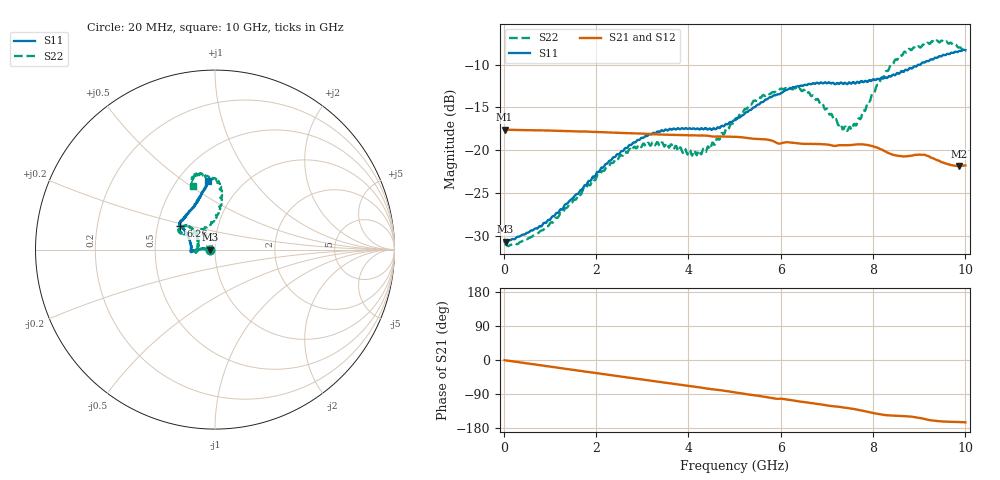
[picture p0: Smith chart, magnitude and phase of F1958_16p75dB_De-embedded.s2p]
! Integrated Device Technology
! Corporate Headquarters
! 6024 Silver Creek Valley Road
! San Jose, CA 95138  USA
! Phone:  1-408-284-8200
! Toll Free:  1-800-223-1366
! Webpage:  http://www.idt.com/
! Timing and RF Division
! 515 Groton Road, Suite 102
! Westford, MA 01886-6024
! Device:  F1958
! Description: 7-bit 0.25 dB Digital Step Attenuator
! Frequency:  0.001 -  6.000 GHz
! Package:  4x4 mm Thin QFN Plastic Package: 24 pin
! Ports:  2 RF, 12 DC
!  Pin  1  = D0
!  Pin  2  = VDD
!  Pin  3  = VMODE
!  Pin  4  = GND
!  Pin  5  = RF1  =  Port 1
!  Pin  6  = GND
!  Pin  7  = GND
!  Pin  8  = GND
!  Pin  9  = GND
!  Pin 10  = GND
!  Pin 11  = GND
!  Pin 12  = GND
!  Pin 13  = GND
!  Pin 14  = RF2  =  Port 2
!  Pin 15  = GND
!  Pin 16  = LE
!  Pin 17  = CLK
!  Pin 18  = DATA
!  Pin 19  = D6
!  Pin 20  = D5
!  Pin 21  = D4
!  Pin 22  = D3
!  Pin 23  = D2
!  Pin 24  = D1
! State:  67
! Atten State:  16.75 dB
! Voltage:  +3.30 Volts
! Current:  0.258 mA
! Data:  The device was measured on a F1958 evaluation board which has
!  individual transmission lines to the RF pins.  Data was collected
!  using a calibrated network analyzer.  The evaluation board was
!  de-embedded using Automatic Fixture Removal (AFR).
!  The reference plane is the edge of the package pin.
! Misc:
!  Action Tracker AT0419
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# GHz S dB R 50
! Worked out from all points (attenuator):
!   500 points, 20 MHz to 10 GHz, reference 50 ohm
!   highest |S21| = -17.58 dB at 20 MHz (marker M1); lowest = -21.8 dB at 9.86 GHz (marker M2)
!   lowest |S11| = -30.6 dB at 40 MHz (marker M3), VSWR 1.06, Z = 47.1 - j0.0698 ohm
!   |S11| at or under -10 dB: start of sweep to 9.027 GHz
!   |S22| runs from -31.1 to -7.2 dB; largest |S21 - S12| = 0.00044
!   S11 on the Smith chart (normalised r, x): 20 MHz: 0.94, -0.00; 6.26 GHz: 0.66, +0.18; 10 GHz: 0.69, +0.62
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0.02  -30.61 -178.5  -17.58 -0.5  -17.57 -0.4  -30.98 -178.7
0.04  -30.64 -178.6  -17.59 -0.8  -17.58 -0.8  -30.94 -178.2
0.32  -30.04 177.5  -17.62 -5.7  -17.62 -5.7  -30.84 177.1
0.84  -28.68 175.6  -17.67 -14.6  -17.67 -14.6  -29.30 176.6
1.7  -24.55 176.3  -17.80 -29.3  -17.79 -29.3  -24.78 175.4
2.62  -19.80 -179.8  -17.98 -44.9  -17.96 -45.0  -20.17 -178.4
2.92  -18.77 -177.1  -18.03 -50.0  -18.02 -50.1  -19.35 -175.8
3.36  -17.85 -174.7  -18.14 -57.6  -18.14 -57.7  -19.33 -171.4
4.24  -17.57 -179.9  -18.26 -72.3  -18.27 -72.3  -20.04 166.7
4.5  -17.61 174.2  -18.37 -77.0  -18.38 -77.1  -19.42 151.5
5.02  -16.47 159.9  -18.42 -85.7  -18.43 -85.7  -16.28 138.5
5.54  -14.62 149.8  -18.67 -94.9  -18.68 -94.9  -13.85 139.8
6.26  -12.65 145.8  -19.11 -106.9  -19.12 -106.9  -12.90 150.6
6.68  -12.22 143.7  -19.25 -113.7  -19.26 -113.6  -13.65 153.0
7.3  -12.09 137.2  -19.39 -124.2  -19.40 -124.0  -16.91 132.2
7.5  -12.13 134.3  -19.39 -127.7  -19.39 -127.6  -17.25 114.3
7.7  -12.16 130.2  -19.29 -132.0  -19.29 -132.0  -16.25 98.0
8.34  -11.36 115.3  -20.31 -146.2  -20.32 -146.3  -10.59 82.6
8.68  -10.74 108.6  -20.69 -148.2  -20.69 -148.1  -8.49 87.0
9.26  -9.37 100.8  -20.85 -159.2  -20.85 -159.2  -7.38 99.6
9.86  -8.44 96.2  -21.82 -163.6  -21.85 -163.6  -8.03 108.2
10  -8.33 96.1  -21.74 -164.6  -21.79 -164.4  -8.52 108.8
